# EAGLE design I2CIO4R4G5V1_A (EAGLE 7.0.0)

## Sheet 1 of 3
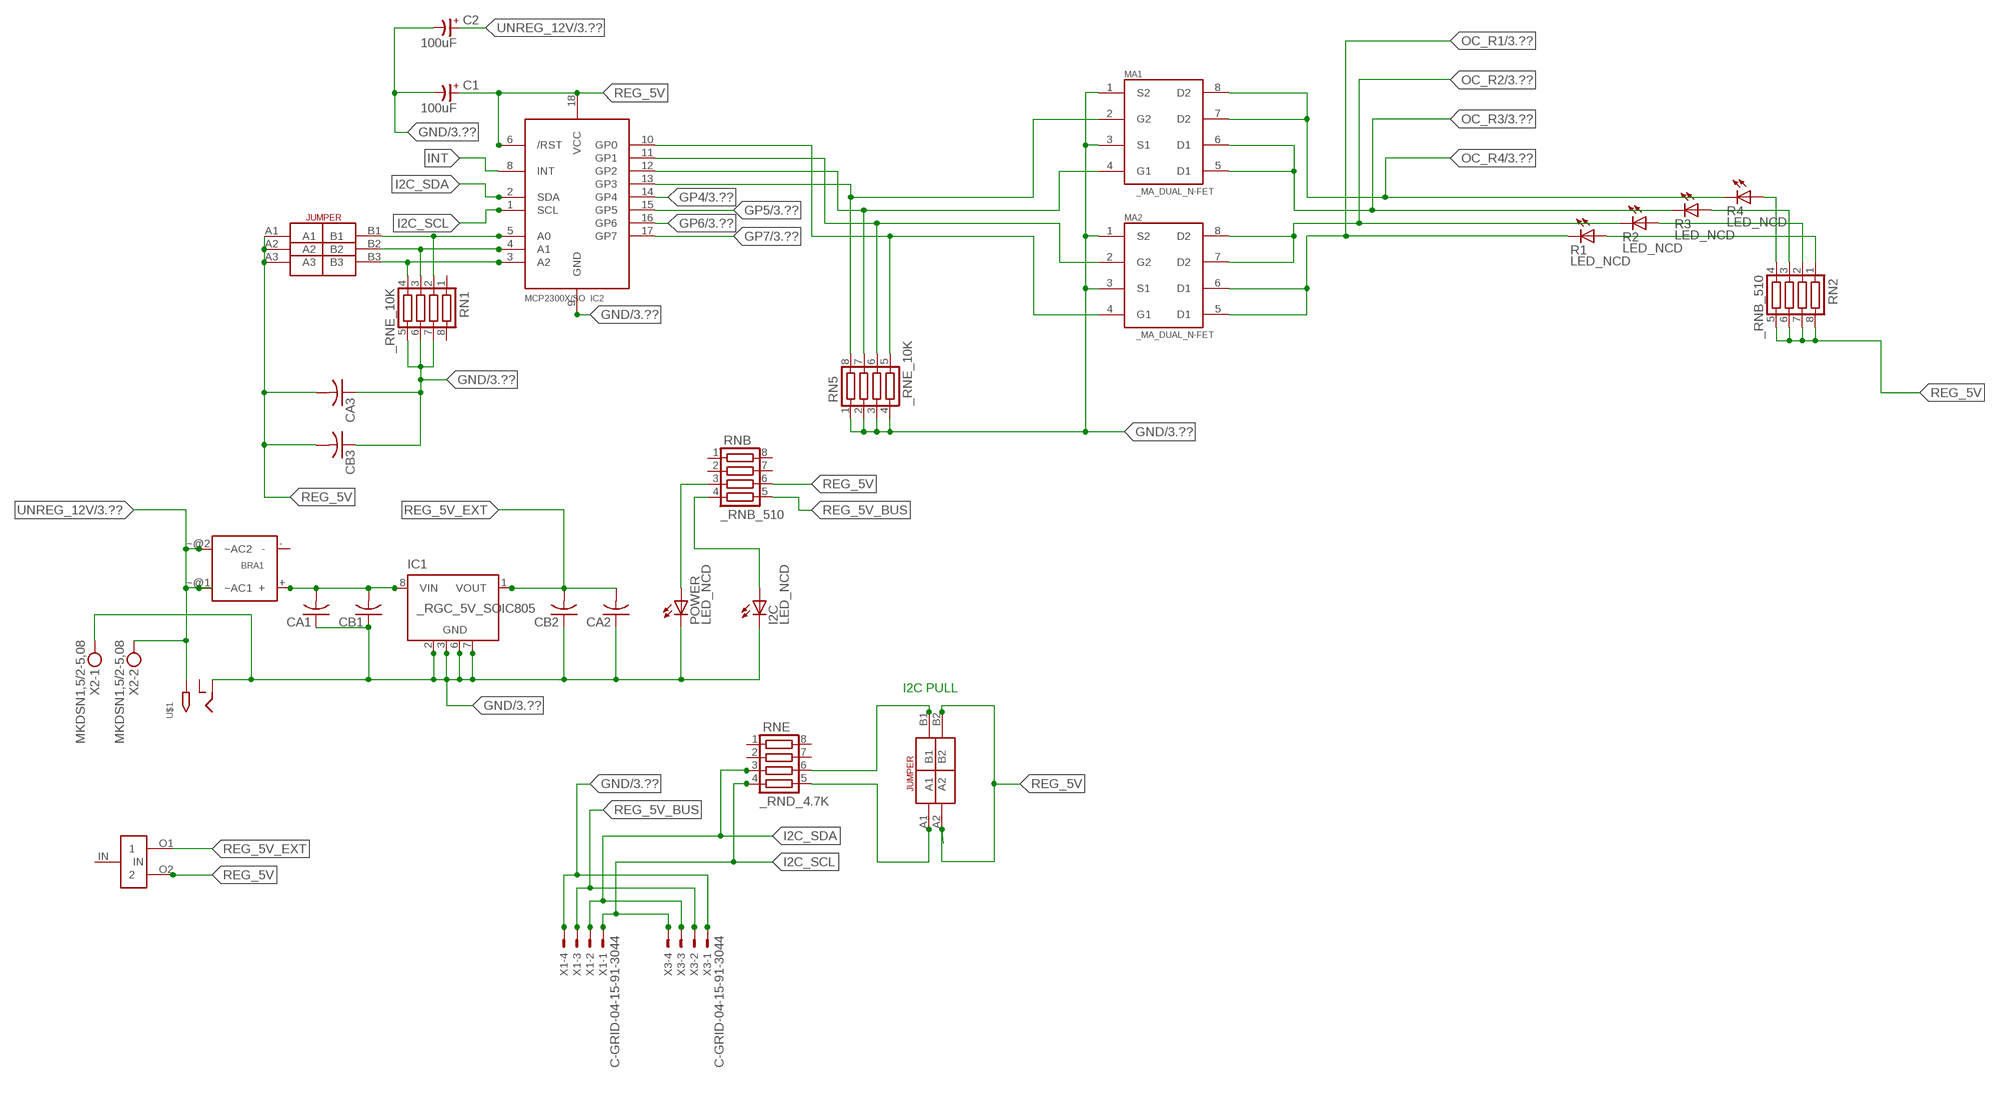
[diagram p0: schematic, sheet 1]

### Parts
BRA1  MB2S_  [MB2S]
C1  100uF  CP-E-025X060  [E-025X060]
C2  100uF  CP-E-025X060  [E-025X060]
CA1  CC1206KRX7R9BB104C1206K  [CC1206KRX7R9BB104]
CA2  CC1206KRX7R9BB104C1206K  [CC1206KRX7R9BB104]
CA3  CC1206KRX7R9BB104C1206K  [CC1206KRX7R9BB104]
CB1  TMK316F106ZL-TC1206K  [TMK316F106ZL-T]
CB2  TMK316F106ZL-TC1206K  [TMK316F106ZL-T]
CB3  TMK316F106ZL-TC1206K  [TMK316F106ZL-T]
I2C  LED_NCD  [CHIPLED_0603]
IC1  _RGC_5V_SOIC805  [_RGC_5V_SOIC8]
IC2  MCP2300X/SO  [SO18W]
MA1  _MA_DUAL_N-FET  [_MA_DUAL_N-FET]
MA2  _MA_DUAL_N-FET  [_MA_DUAL_N-FET]
POWER  LED_NCD  [CHIPLED_0603]
R1  LED_NCD  [CHIPLED_0603]
R2  LED_NCD  [CHIPLED_0603]
R3  LED_NCD  [CHIPLED_0603]
R4  LED_NCD  [CHIPLED_0603]
RN1  _RNE_10K  [RNE]
RN2  _RNB_510  [RNB]
RN5  _RNE_10K  [RNE]
RNB  _RNB_510  [RNB]
RNE  _RND_4.7K  [RND]
U$1  2.1MMJACK  [PJ-102A]
U$3  JUMPER_2X2  [JUMPER_2X2]
U$5  LINK_2  [LINK_2]
U$18  JUMPER_3X2  [JUMPER_3X2]
X1  C-GRID-04-15-91-3044  [15-91-04]
X2  MKDSN1,5/2-5,08  [MKDSN1,5/2-5,08]
X3  C-GRID-04-15-91-3044  [15-91-04]

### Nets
GND: C1.- C2.- CA1.1 CA2.1 CA3.1 CB1.1 CB2.1 CB3.1 I2C.C IC1.2(GND) IC1.3(GND) IC1.6(GND) IC1.7(GND) IC2.9(GND) MA1.1(S2) MA1.3(S1) MA2.1(S2) MA2.3(S1) POWER.C RN1.5 RN1.6 RN1.7 RN5.1 RN5.2 RN5.3 RN5.4 U$1.RING X1.4 X2.1 X3.1 ; also sheet 3
GP4: IC2.14(GP4) ; also sheet 3
GP5: IC2.15(GP5) ; also sheet 3
GP6: IC2.16(GP6) ; also sheet 3
GP7: IC2.17(GP7) ; also sheet 3
I2C_SCL: IC2.1(SCL) RNE.4 X1.1 X3.4
I2C_SDA: IC2.2(SDA) RNE.3 X1.2 X3.3
INT: IC2.8(INT)
N$1: BRA1.+ CA1.2 CB1.2 IC1.8(VIN)
N$2: POWER.A RNB.3
N$3: I2C.A RNB.4
N$4: RNE.5 U$3.A1
N$5: RNE.6 U$3.B1
N$6: IC2.5(A0) RN1.2 U$18.B1
N$7: IC2.4(A1) RN1.3 U$18.B2
N$8: IC2.3(A2) RN1.4 U$18.B3
N$20: IC2.13(GP3) MA1.2(G2) RN5.8
N$21: IC2.12(GP2) MA1.4(G1) RN5.7
N$22: IC2.11(GP1) MA2.2(G2) RN5.6
N$23: IC2.10(GP0) MA2.4(G1) RN5.5
N$29: R4.A RN2.4
N$30: R3.A RN2.3
N$31: R2.A RN2.2
N$32: R1.A RN2.1
OC_R1: MA2.5(D1) MA2.6(D1) R1.C ; also sheet 3
OC_R2: MA2.7(D2) MA2.8(D2) R2.C ; also sheet 3
OC_R3: MA1.5(D1) MA1.6(D1) R3.C ; also sheet 3
OC_R4: MA1.7(D2) MA1.8(D2) R4.C ; also sheet 3
REG_5V: C1.+ CA3.2 CB3.2 IC2.6(/RST) IC2.18(VCC) RN2.5 RN2.6 RN2.7 RN2.8 RNB.6 U$3.A2 U$3.B2 U$5.O2 U$18.A1 U$18.A2 U$18.A3
REG_5V_BUS: RNB.5 X1.3 X3.2
REG_5V_EXT: CA2.2 CB2.2 IC1.1(VOUT) U$5.O1
UNREG_12V: BRA1.~@1(~AC1) BRA1.~@2(~AC2) C2.+ U$1.TIP X2.2 ; also sheet 3
Unconnected: BRA1.- IC1.4(NC) IC1.5(NC) RN1.1 RN1.8 RNB.1 RNB.2 RNB.7 RNB.8 RNE.1 RNE.2 RNE.7 RNE.8 U$1.RING_SW U$5.IN

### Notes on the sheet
- I2C PULL

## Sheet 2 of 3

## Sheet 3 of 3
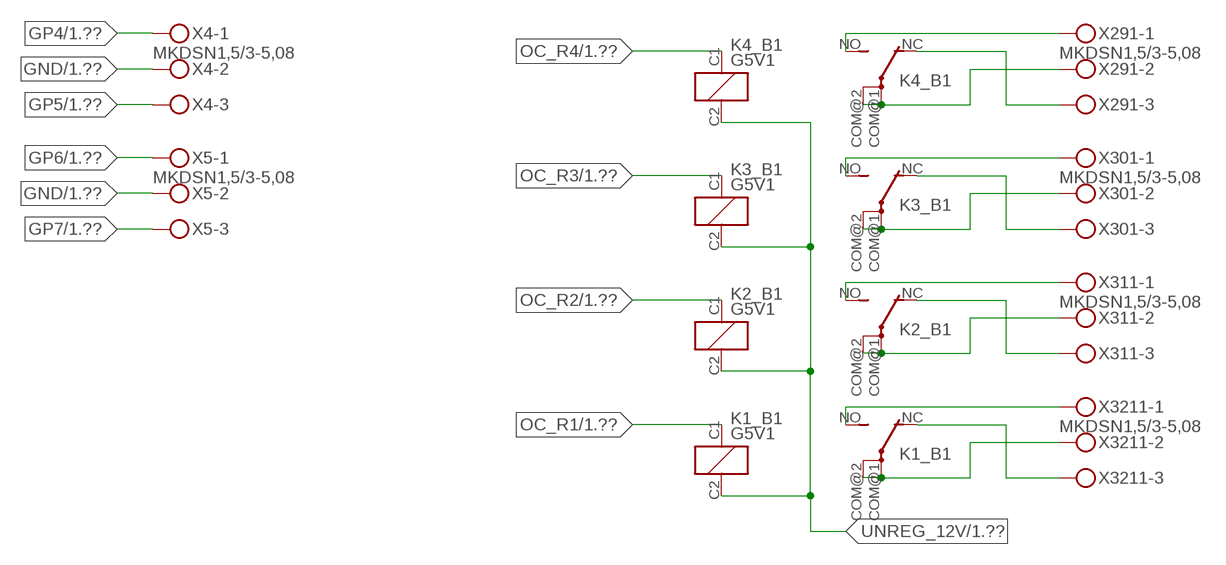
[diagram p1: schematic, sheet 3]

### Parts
K1_B1  G5V1  [G5V1]
K2_B1  G5V1  [G5V1]
K3_B1  G5V1  [G5V1]
K4_B1  G5V1  [G5V1]
X4  MKDSN1,5/3-5,08  [MKDSN1,5/3-5,08]
X5  MKDSN1,5/3-5,08  [MKDSN1,5/3-5,08]
X291  MKDSN1,5/3-5,08  [MKDSN1,5/3-5,08]
X301  MKDSN1,5/3-5,08  [MKDSN1,5/3-5,08]
X311  MKDSN1,5/3-5,08  [MKDSN1,5/3-5,08]
X3211  MKDSN1,5/3-5,08  [MKDSN1,5/3-5,08]

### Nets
GND: X4.2 X5.2 ; also sheet 1
GP4: X4.1 ; also sheet 1
GP5: X4.3 ; also sheet 1
GP6: X5.1 ; also sheet 1
GP7: X5.3 ; also sheet 1
N$215: K4_B1.NO(2:S) X291.1
N$216: K4_B1.NC(2:O) X291.3
N$217: K4_B1.COM@1(2:P) K4_B1.COM@2(2:P) X291.2
N$218: K3_B1.NO(2:S) X301.1
N$219: K3_B1.NC(2:O) X301.3
N$220: K3_B1.COM@1(2:P) K3_B1.COM@2(2:P) X301.2
N$221: K2_B1.NO(2:S) X311.1
N$222: K2_B1.NC(2:O) X311.3
N$223: K2_B1.COM@1(2:P) K2_B1.COM@2(2:P) X311.2
N$224: K1_B1.NO(2:S) X3211.1
N$225: K1_B1.NC(2:O) X3211.3
N$226: K1_B1.COM@1(2:P) K1_B1.COM@2(2:P) X3211.2
OC_R1: K1_B1.C1(1:C1) ; also sheet 1
OC_R2: K2_B1.C1(1:C1) ; also sheet 1
OC_R3: K3_B1.C1(1:C1) ; also sheet 1
OC_R4: K4_B1.C1(1:C1) ; also sheet 1
UNREG_12V: K1_B1.C2(1:C2) K2_B1.C2(1:C2) K3_B1.C2(1:C2) K4_B1.C2(1:C2) ; also sheet 1

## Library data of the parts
BRA1 = NCD_ULTIMATE_LIBRARY:MB2S: Bridge Rectifier BRA MB2S 200V 500ma Digikey MB2S-TPMSTR-ND/MB2S-TP
C1 C2 = NCD_ULTIMATE_LIBRARY:CP-: Capacitors All Kinds POLARIZED CAP
CA1-CA3 = NCD_ULTIMATE_LIBRARY:CC1206KRX7R9BB104: Capacitor CA .1uF 50V SMT C1206K CC1206KRX7R9BB104
CB1-CB3 = NCD_ULTIMATE_LIBRARY:TMK316F106ZL-T: Capacitor CB 10uF SMT 1206 TMK316F106ZL-T
I2C POWER = NCD_ULTIMATE_bhaskar:LED_NCD
IC1 = NCD_ULTIMATE_LIBRARY:_RGC_5V_SOIC8: Regulator Linear 5V Chip Positive VOLTAGE REGULATOR Digikey 497-7267-2-ND/L78L05CD13TR
IC2 = NCD_ULTIMATE_LIBRARY:MCP2300X: Semiconductor Port Expander I/O 8-Bit I2C MCP23008 Inexpensive i2c i/o expander - 8 general purpose i/o pins with optional pullups
K1_B1 K2_B1 K3_B1 K4_B1 = NCD_ULTIMATE_LIBRARY:G5V1: RELAY 1 x switch, 0.5 A/125 V AC, 1 A/24 V DC , Omron
MA1 MA2 = NCD_ULTIMATE_LIBRARY:_MA_DUAL_N-FET: FET Dual N-Channel 8-SOIC NMOSFET Digikey 785-1064-2-ND/AO4842
R1-R4 = NCD_ULTIMATE_LIBRARY:LED_NCD: LED Digikey 754-1132-2-ND/APT2012SRCPRV
RN1 RN5 = NCD_ULTIMATE_LIBRARY:_RNE_10K: Resistor Array RNE SMT 10K x 4 Single Resistor Source: http://www.ctscorp.com/components/Datasheets/CTSChipArrayDs.pdf Digikey 742C083103JPTR-ND/742C083103JP; OC_FARNELL: unknown; OC_NEWARK: unknown
RN2 RNB = NCD_ULTIMATE_LIBRARY:_RNB_510: Resistor Array RNB SMT 510 x 4 Single Resistor Source: http://www.ctscorp.com/components/Datasheets/CTSChipArrayDs.pdf Digikey 742C083511JPTR-ND/ 742C083511JP; OC_FARNELL: unknown; OC_NEWARK: unknown
RNE = NCD_ULTIMATE_LIBRARY:_RND_4.7K: Resistor Array RND SMT 4.7K x 4 Single Resistor Source: http://www.ctscorp.com/components/Datasheets/CTSChipArrayDs.pdf Digikey 742C083472JPTR-ND/742C083472JP; OC_FARNELL: unknown; OC_NEWARK: unknown
U$1 = NCD_ULTIMATE_CONNECTORS:2.1MMJACK: 2.1mm x 5.5mm DC jack with internal switch. Digikey part #PJ-102A, 4UCON part #05537 By microbuilder.eu
U$3 = NCD_ULTIMATE_CONNECTORS:JUMPER_2X2
U$5 = NCD_ULTIMATE_LIBRARY:LINK_2: PAD_top
U$18 = NCD_ULTIMATE_CONNECTORS:JUMPER_3X2
X1 X3 = NCD_ULTIMATE_CONNECTORS:C-GRID-04: CONNECTOR 4-Pos I2C wire to board 2.54 mm (0.100") pitch header Digikey WM1342-ND/0015912045; OC_FARNELL: unknown; OC_NEWARK: unknown
X2 = NCD_ULTIMATE_CONNECTORS:MKDSN1,5/2-5,08: MKDSN 1,5/ 2-5,08 Printklemme
X4 X5 X291 X301 X311 X3211 = NCD_ULTIMATE_CONNECTORS:MKDSN1,5/3-5,08: MKDSN 1,5/ 3-5,08 Printklemme Nennstrom: 13,5 A Nennspannung: 250 V Rastermaß: 5,08 mm Polzahl: 3 Anschlussart: Schraubanschluss Montage: Löten Anschlussrichtung Leiter/Platine: 0 ° Artikelnummer: 1729131 Source: http://eshop.phoenixcontact.com .. 1729131.pdf

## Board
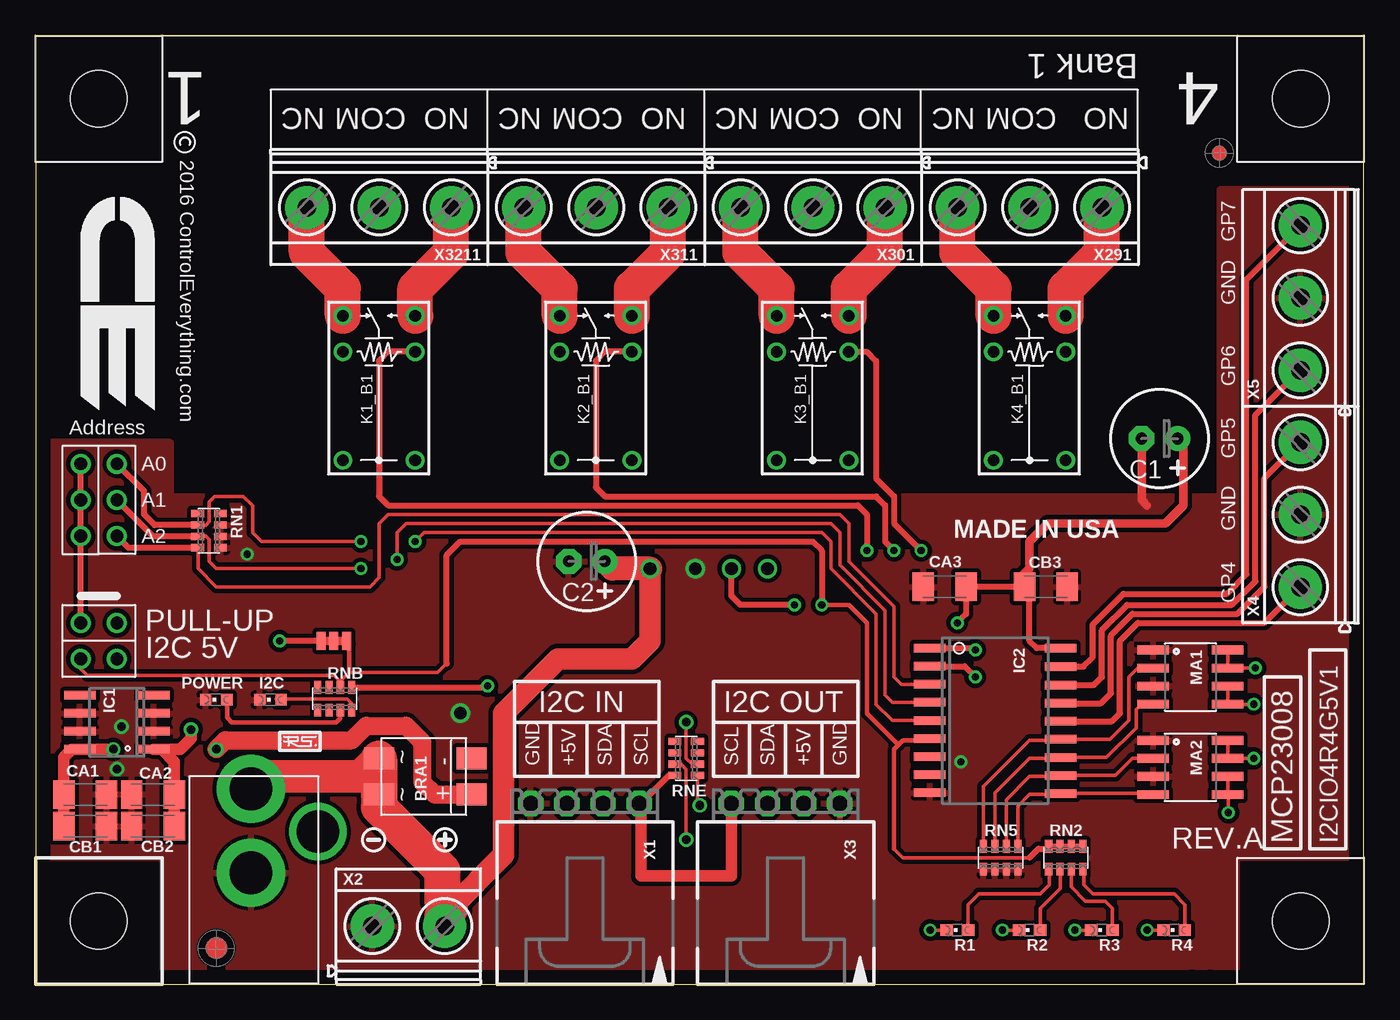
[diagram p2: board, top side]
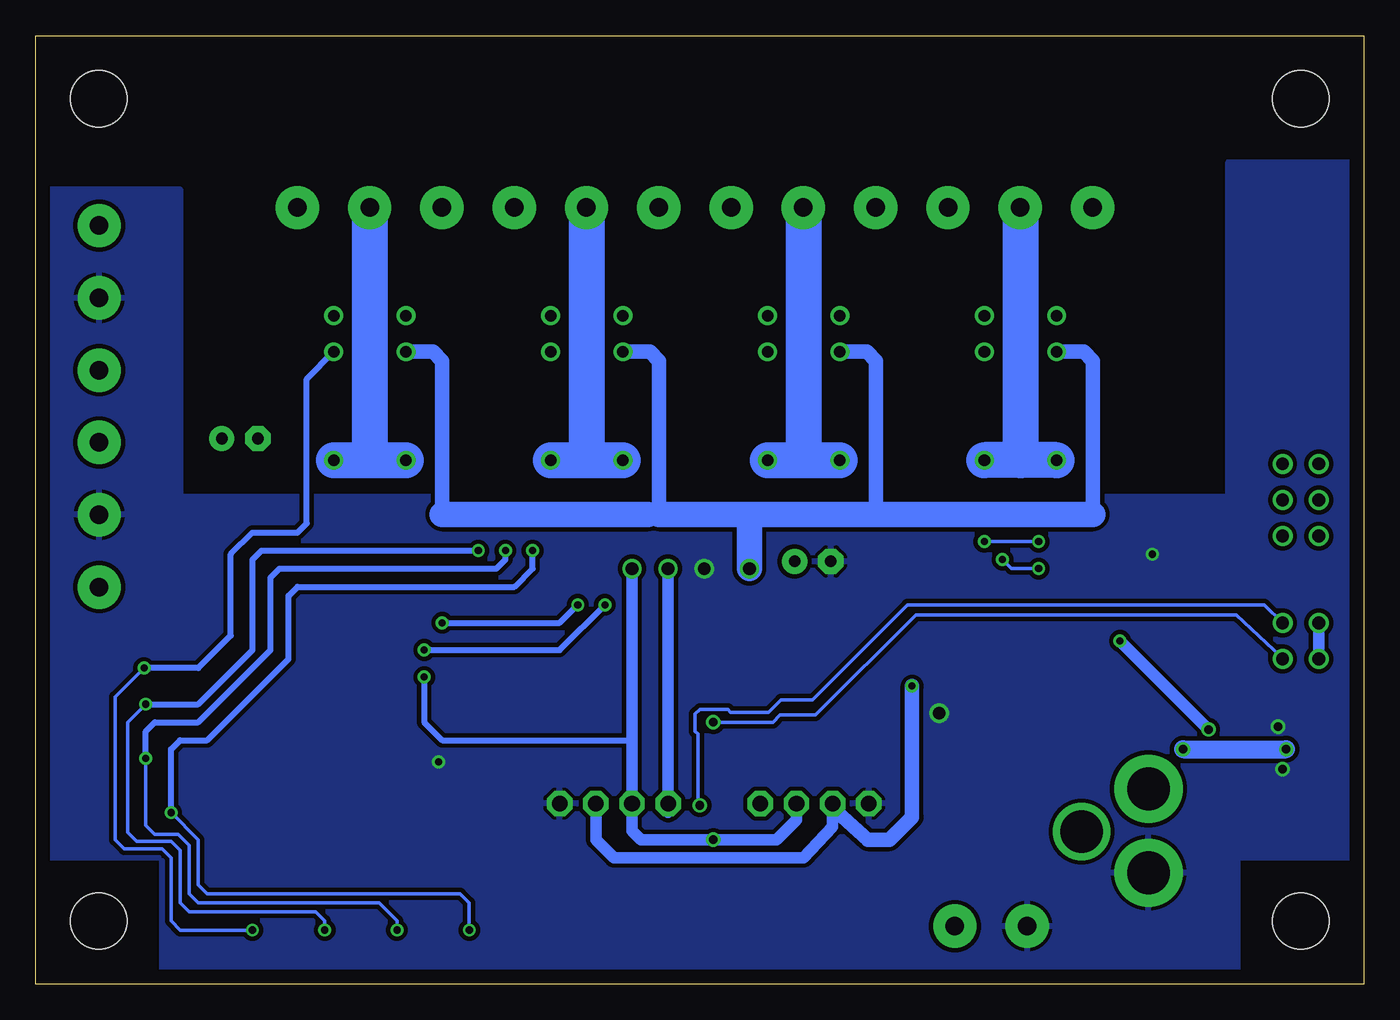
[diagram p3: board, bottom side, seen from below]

Size 93.34 x 66.67 mm. Coordinates in mm from the lower left corner, seen from the top.
Outline: 81.28,0 0,0 0,46.35
Outline: 81.28,0 82.53,0
Outline: 0,47.3 0,46.35
Outline: 81.28,0 93.34,0 93.34,66.67 0,66.67 0,46.35
Copper layers (1*16): Top 0.035mm / dielectric 1.5mm / Bottom 0.035mm
Design rules "default": minimum track width 10mil, minimum drill 24mil, track to track 8mil, track to pad 8mil, pad to pad 8mil, via to via 8mil, smd to smd 8mil, copper to edge 40mil, drill to drill 8mil, minimum pad ring 10mil, minimum via ring 8mil, stop-mask expansion 4mil, vias tented up to drill 0mil, thermal gap 10mil
Holes 3.96 mm at 4.45,4.45

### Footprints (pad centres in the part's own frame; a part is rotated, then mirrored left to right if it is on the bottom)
MB2S = smd 1.55 x 2.1: + 0,-6.5; - 2.54,-6.5; ~@1 0,0; ~@2 2.54,0
E-025X060 = drill 0.813 pad 1.778: + -1.27,0 | drill 0.813 pad 1.778 octagon: - 1.27,0
CC1206KRX7R9BB104 = smd 1.5 x 2: 1 -1.5,0; 2 1.5,0
TMK316F106ZL-T = smd 1.5 x 2: 1 -1.5,0; 2 1.5,0
CHIPLED_0603 = smd 0.8 x 0.8: A 0,-0.75; C 0,0.75
_RGC_5V_SOIC8 = smd 0.6 x 2.2: 1 -1.905,-2.6; 2 -0.635,-2.6; 3 0.635,-2.6; 4 1.905,-2.6; 5 1.905,2.6; 6 0.635,2.6; 7 -0.635,2.6; 8 -1.905,2.6
SO18W = smd 0.6 x 2.2: 1 -4.445,-4.6; 2 -3.175,-4.6; 3 -1.905,-4.6; 4 -0.635,-4.6; 5 0.635,-4.6; 6 1.905,-4.6; 7 3.175,-4.6; 8 4.445,-4.6; 9 5.715,-4.6; 10 5.775,4.6; 11 4.505,4.6; 12 3.235,4.6; 13 1.965,4.6; 14 0.695,4.6; 15 -0.575,4.6; 16 -1.845,4.6; 17 -3.145,4.6; 18 -4.445,4.6
G5V1 = drill 0.813: C1 -2.54,2.54; C2 -2.54,-2.54; COM@1 5.08,-2.54; COM@2 5.08,2.54; NC -5.08,-2.54; NO -5.08,2.54
_MA_DUAL_N-FET = smd 0.61 x 2.21: 1 -1.905,-2.616; 2 -0.635,-2.616; 3 0.635,-2.616; 4 1.905,-2.616; 5 1.905,2.616; 6 0.635,2.616; 7 -0.635,2.616; 8 -1.905,2.616
CHIPLED_0603' = smd 0.8 x 0.876: A 0,-0.75; C 0,0.75
RNE = smd 0.5 x 0.9: 1 -1.2,-0.8; 2 -0.4,-0.8; 3 0.4,-0.8; 4 1.2,-0.8; 5 1.2,0.8; 6 0.4,0.8; 7 -0.4,0.8; 8 -1.2,0.8
RNB = smd 0.5 x 0.9: 1 -1.2,-0.8; 2 -0.4,-0.8; 3 0.4,-0.8; 4 1.2,-0.8; 5 1.2,0.8; 6 0.4,0.8; 7 -0.4,0.8; 8 -1.2,0.8
RND = smd 0.5 x 0.9: 1 -1.2,-0.8; 2 -0.4,-0.8; 3 0.4,-0.8; 4 1.2,-0.8; 5 1.2,0.8; 6 0.4,0.8; 7 -0.4,0.8; 8 -1.2,0.8
PJ-102A = drill 3 pad 4.8: RING 0.1,-3.39; TIP 0.1,-9.29 | drill 3 pad 3.251: RING_SW -4.6,-6.29
JUMPER_2X2 = drill 0.9: A1 0,2.54; A2 0,0; B1 2.54,2.54; B2 2.54,0
PCB_MOUNTING_HOLE = hole 3.962: 4.445,4.445
LINK_2 = smd 1.27 x 0.635: IN 0,0; O1 0,0.889; O2 0,-0.889
JUMPER_3X2 = drill 0.9: A1 0,5.08; A2 0,2.54; A3 0,0; B1 2.54,5.08; B2 2.54,2.54; B3 2.54,0
15-91-04 = drill 1.1 pad 1.778 octagon: 1 -3.81,-7.62; 2 -1.27,-7.62; 3 1.27,-7.62; 4 3.81,-7.62
MKDSN1,5/2-5,08 = drill 1.3 pad 3.048: 1 -2.561,0.025; 2 2.519,0.025
MKDSN1,5/3-5,08 = drill 1.3 pad 3.048: 1 -7.641,0.025; 2 -2.561,0.025; 3 2.519,0.025

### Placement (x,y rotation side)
BRA1  24.13,13.34 90 top
C1  78.99,38.35 180 top
C2  38.73,29.72 180 top
CA1  3.49,13.34 180 top
CA2  8.26,13.34 0 top
CA3  63.88,27.94 0 top
CB1  3.49,11.11 180 top
CB2  8.26,11.11 0 top
CB3  70.99,27.94 180 top
I2C  16.51,20 90 top
IC1  5.71,18.41 90 top
IC2  67.44,19.18 270 top
K1_B1  24.13,41.91 270 top
K2_B1  39.37,41.91 270 top
K3_B1  54.61,41.91 270 top
K4_B1  69.85,41.91 270 top
MA1  81.15,21.59 270 top
MA2  81.15,15.24 270 top
POWER  12.7,20 90 top
R1  LED_NCD  [CHIPLED_0603']  64.77,3.81 90 top
R2  LED_NCD  [CHIPLED_0603']  69.85,3.81 90 top
R3  LED_NCD  [CHIPLED_0603']  74.93,3.81 90 top
R4  LED_NCD  [CHIPLED_0603']  80.01,3.81 90 top
RN1  12.19,31.88 270 top
RN2  72.39,8.89 0 top
RN5  67.82,8.89 0 top
RNB  21.02,20.07 0 top
RNE  45.72,15.88 270 top
U$1  15.24,4.45 180 top
U$3  3.17,25.4 270 top
U$4  PCB_MOUNTING_HOLE  [PCB_MOUNTING_HOLE]  93.34,57.78 90 top
U$5  20.95,24.13 90 top
U$6  PCB_MOUNTING_HOLE  [PCB_MOUNTING_HOLE]  93.34,0 90 top
U$10  [VISION_REF15]  12.7,2.54 0 top
U$11  PCB_MOUNTING_HOLE  [PCB_MOUNTING_HOLE]  8.89,57.78 90 top
U$18  3.17,31.5 0 top
U$19  [VISION_REF10]  83.19,58.42 0 top
U$21  [ICON_USA]  64.52,31.37 0 top
U$22  [ICON_MINUS]  23.75,10.16 180 top
U$24  [ICON_PLUS]  28.77,10.16 90 top
X1  38.61,5.08 180 top
X2  26.23,4.06 0 top
X3  52.7,5.08 180 top
X4  88.9,35.56 90 top
X5  88.9,50.8 90 top
X291  67.31,54.61 180 top
X301  52.07,54.61 180 top
X311  36.83,54.61 180 top
X3211  21.59,54.61 180 top

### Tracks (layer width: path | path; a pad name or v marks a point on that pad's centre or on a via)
GND  (via drill 0.5, 0.6, 0.9)
  Top 0.406: 34.8,12.38 X1.4
  Top 0.61: C1.- 77.72,34.04 78.11,33.66
  Top 0.813: X3.1 56.52,12.06
  other vias: 5.71,15.11 6.03,18.1 46.35,29.21 29.84,19.05 14.86,30.23 65.02,15.62
  pour Bottom (isolate 0.305): 0.64,8.89 8.89,8.89 8.89,0 84.45,0 84.45,8.89 92.71,8.89 92.71,55.88 83.19,55.88 83.19,34.29 9.53,34.29 9.53,57.78 0.64,57.78
  pour Top (isolate 0.305): -1.91,8.89 8.89,8.89 8.89,0 84.45,0 84.45,8.89 92.71,8.89 92.71,55.88 83.19,55.88 83.19,34.29 9.53,34.29 9.53,38.1 -1.91,38.1
GP4
  Top 0.406: IC2.14 75.63,18.48 76.2,19.05 76.2,24.13 77.47,25.4 86.36,25.4 X4.1
GP5
  Top 0.406: IC2.15 74.87,19.75 75.56,20.45 75.56,24.51 77.09,26.04 84.45,26.04 86.36,27.94 86.36,35.56 X4.3
GP6
  Top 0.406: IC2.16 74.36,21.02 74.93,21.59 74.93,24.89 76.71,26.67 84.07,26.67 85.72,28.32 85.72,40.01 X5.1
GP7
  Top 0.406: IC2.17 73.63,22.32 74.3,22.99 74.3,25.27 76.45,27.43 83.69,27.43 85.09,28.83 85.09,49.53 X5.3
I2C_SCL  (via drill 0.5, 0.9)
  Top 0.406: RNE.4 44.51,14.68 42.55,12.7 | IC2.1 65.91,23.62 v66.04,23.5 | v53.34,26.67 49.53,26.67 48.9,27.3 v48.9,29.21
  Top 0.813: X3.4 48.9,7.62 42.55,7.62 42.55,12.7 X1.1
  Bottom 0.406: v66.04,23.5 56.52,23.5 v53.34,26.67
  Bottom 0.813: v48.9,29.21 X3.4 48.9,12.06
I2C_SDA  (via drill 0.5, 0.6, 0.9)
  Top 0.254: RNE.3 45.36,15.47 45.72,15.11 v45.72,10.16
  Top 0.406: IC2.2 65.28,22.35 v66.04,21.59
  Top 0.61: X3.3 51.44,12.06 | X1.2 39.88,12.38
  Bottom 0.406: v66.04,21.59 66.04,18.41 64.77,17.14 51.44,17.14 | 39.88,12.38 X1.2
  Bottom 0.813: 39.88,12.38 39.88,11.56 41.27,10.16 v45.72,10.16 50.8,10.16 51.44,10.79 X3.3 51.44,17.14 v51.44,29.21
N$1  (via drill 0.6)
  Top 0.813: CB1.2 CA1.2 1.99,15.96 2.54,16.51 IC1.8 v5.46,16.51
  Top 1.27: v12.7,16.51 13.34,17.14 22.23,17.14 23.24,18.16 26.04,18.16 27.18,17.02 27.18,14.22 28.07,13.34 BRA1.+
  Bottom 1.27: v12.7,16.51 v5.46,16.51
N$2
  Top 0.305: RNB.3 21.4,18.95 21.4,18.7 21.12,18.41 13.78,18.41 13.45,18.74 POWER.A
N$3
  Top 0.254: 22.23,18.95 22.23,19.74 21.9,20.07 16.94,20.07
  Top 0.305: RNB.4 22.23,18.95 | 16.94,20.07 I2C.A
N$4  (via drill 0.6)
  Top 0.254: RNE.5 46.52,12.6 v46.67,12.57
  Bottom 0.254: U$3.A1 6.99,26.67 32.07,26.67 38.73,20 40.96,20 41.85,19.11 44.51,19.11 44.7,19.3 46.67,19.3 46.99,18.99 46.99,17.78 46.8,17.59 46.8,12.7 v46.67,12.57
N$5  (via drill 0.6)
  Top 0.254: RNE.6 46.12,15.47 45.72,15.88 v45.72,18.41
  Bottom 0.254: v45.72,18.41 41.53,18.41 41.02,18.92 38.54,18.92 31.5,25.97 8.95,25.97 6.35,23.5 U$3.B1
N$6  (via drill 0.5)
  Top 0.254: IC2.5 60.2,18.54 59.05,19.68 59.05,26.04 55.88,29.21 55.88,31.11 55.24,31.75 27.3,31.75 v26.67,31.11 | v22.86,31.11 15.88,31.11 15.24,31.75 15.24,33.66 14.61,34.29 12.57,34.29 12.19,33.91 12.19,32.51 11.94,32.26 11.41,32.26 RN1.2
  Top 0.406: RN1.2 8.36,32.28 7.62,33.02 7.62,34.67 U$18.B1
  Bottom 0.254: v26.67,31.11 v22.86,31.11
N$7  (via drill 0.5)
  Top 0.254: IC2.4 60.2,19.81 59.69,20.32 59.69,26.29 56.52,29.46 56.52,31.75 55.88,32.38 26.04,32.38 25.4,31.75 v25.4,29.84 | v22.86,29.21 12.7,29.21 12.19,29.72 12.19,31.24 11.94,31.5 11.41,31.5 RN1.3
  Top 0.406: RN1.3 8.27,31.48 U$18.B2
  Bottom 0.254: v25.4,29.84 24.77,29.21 v22.86,29.21
N$8
  Top 0.254: IC2.3 60.83,21.08 60.33,21.59 60.33,26.54 57.15,29.72 57.15,32.38 56.52,33.02 24.77,33.02 24.13,32.38 24.13,28.57 23.5,27.94 12.7,27.94 11.43,29.21 11.43,30.64 RN1.4
  Top 0.406: RN1.4 6.53,30.68 U$18.B3
N$20
  Top 0.254: MA1.2 77.47,22.23 76.83,21.59 76.83,18.54 75.5,17.21 IC2.13 71.97,17.14 69.85,17.14 66.62,13.91 RN5.8
N$21
  Top 0.254: MA1.4 77.72,19.68 77.34,19.3 77.34,18.03 75.25,15.94 IC2.12 71.97,15.88 69.85,15.88 67.42,13.44 RN5.7
N$22
  Top 0.254: MA2.2 77.09,15.88 75.89,14.67 IC2.11 71.97,14.61 69.85,14.61 68.22,12.97 RN5.6
N$23
  Top 0.254: MA2.4 78.6,13.4 IC2.10 71.97,13.34 69.85,13.34 69.02,12.5 RN5.5
N$29
  Top 0.254: R4.A 80.76,5.6 80.01,6.35 74.3,6.35 73.66,6.99 73.66,8.02 RN2.4
N$30
  Top 0.254: R3.A 75.68,5.35 75.18,5.84 73.79,5.84 72.77,6.86 72.77,8.07 RN2.3
N$31
  Top 0.254: R2.A 70.6,5.32 72.01,6.73 72.01,8.07 RN2.2
N$32
  Top 0.254: R1.A 65.52,5.58 66.29,6.35 70.61,6.35 71.25,6.99 71.25,8.03 RN2.1
N$215
  Top 2.54: K4_B1.NO 72.39,48.9 74.93,51.44 74.93,54.56 X291.1
N$216
  Top 2.54: K4_B1.NC 67.31,48.9 64.77,51.44 64.77,54.56 X291.3
N$217
  Bottom 2.54: X291.2 69.87,36.85 | 69.87,36.85 69.85,36.83 K4_B1.COM@1 | K4_B1.COM@2 69.89,36.83 69.87,36.85
N$218
  Top 2.54: K3_B1.NO 57.15,48.9 59.69,51.44 59.69,54.56 X301.1
N$219
  Top 2.54: K3_B1.NC 52.07,48.9 49.53,51.44 49.53,54.56 X301.3
N$220
  Bottom 2.54: K3_B1.COM@2 54.61,36.83 | 54.61,36.83 K3_B1.COM@1 | X301.2 54.63,36.85 54.61,36.83
N$221
  Top 2.54: K2_B1.NO 41.91,48.9 44.45,51.44 44.45,54.56 X311.1
N$222
  Top 2.54: K2_B1.NC 36.83,48.9 34.29,51.44 34.29,54.56 X311.3
N$223
  Bottom 2.54: K2_B1.COM@2 39.37,36.83 | 39.37,36.83 K2_B1.COM@1 | X311.2 39.39,36.85 39.37,36.83
N$224
  Top 2.54: K1_B1.NO 26.67,48.9 29.21,51.44 29.21,54.56 X3211.1
N$225
  Top 2.54: K1_B1.NC 21.59,48.9 19.05,51.44 19.05,54.56 X3211.3
N$226
  Bottom 2.54: K1_B1.COM@1 24.13,36.83 | 24.13,36.83 K1_B1.COM@2 | X3211.2 24.15,36.85 24.13,36.83
OC_R1  (via drill 0.5)
  Top 0.254: R1.C v62.87,3.81 | v83.82,12.06 83.82,13.26 MA2.5 MA2.6
  Top 0.406: v58.42,30.48 58.42,33.02 57.78,33.66 24.77,33.66 24.13,34.29 24.13,43.81 24.77,44.45 K1_B1.C1
  Bottom 0.254: v62.87,3.81 62.87,5.71 63.5,6.35 81.28,6.35 81.92,6.99 81.92,10.16 v83.82,12.06
  Bottom 0.406: v83.82,12.06 83.82,16.51 83.19,17.14 81.28,17.14 75.56,22.86 75.56,27.3 74.93,27.94 59.69,27.94 58.42,29.21 v58.42,30.48
OC_R2  (via drill 0.5)
  Top 0.254: R2.C v67.94,3.81 | v85.6,15.88 MA2.7 MA2.8
  Top 0.406: v60.33,30.48 59.69,31.11 59.69,33.66 59.05,34.29 40.01,34.29 39.37,34.92 39.37,43.81 40.01,44.45 K2_B1.C1
  Bottom 0.254: v67.94,3.81 67.94,4.45 69.22,5.71 81.92,5.71 82.55,6.35 82.55,9.78 83.31,10.54 84.96,10.54 85.6,11.18 v85.6,15.88
  Bottom 0.406: v85.6,15.88 85.6,17.78 84.96,18.41 81.92,18.41 76.83,23.5 76.83,28.57 76.2,29.21 60.96,29.21 60.33,29.84 v60.33,30.48
OC_R3  (via drill 0.5)
  Top 0.254: R3.C v73.03,3.81 | v85.6,19.68 MA1.5 MA1.6
  Top 0.406: 61.85,30.86 v62.23,30.48 60.33,32.38 60.33,34.29 59.05,35.56 59.05,43.81 58.42,44.45 K3_B1.C1
  Bottom 0.254: v73.03,3.81 73.03,4.45 73.66,5.08 82.55,5.08 83.19,5.71 83.19,9.4 83.82,10.03 86.23,10.03 86.87,10.67 86.87,18.41 v85.6,19.68
  Bottom 0.406: v85.6,19.68 81.92,19.68 78.11,23.5 78.11,29.84 77.47,30.48 v62.23,30.48
OC_R4  (via drill 0.5)
  Top 0.254: R4.C v78.11,3.81 | v85.72,22.23 MA1.7 MA1.8
  Bottom 0.254: v78.11,3.81 83.19,3.81 83.82,4.45 83.82,8.89 84.45,9.53 87.12,9.53 87.76,10.16 87.76,20.19 v85.72,22.23
  Bottom 0.406: v85.72,22.23 81.92,22.23 79.63,24.51 79.63,30.23 78.11,31.75 74.93,31.75 74.3,32.38 74.3,42.55 K4_B1.C1
REG_5V  (via drill 0.5)
  Top 0.229: 60.33,9.53 60.96,8.89 69.85,8.89
  Top 0.254: RNB.6 21.42,21.29 | 21.42,21.29 22.04,21.91 28.26,21.91 28.89,22.54 | 21.42,21.29 20.99,21.72 3.62,21.72 3.17,22.16 U$3.B2
  Top 0.305: 62.71,17.14 60.96,17.14 60.64,16.83 | 60.64,16.83 60.33,16.51 60.33,9.53 | 60.64,16.83 58.42,19.05 58.42,25.4 57.15,26.67 v55.24,26.67 | 22.04,21.91 22.04,23.94 U$5.O2
  Top 0.406: U$18.A1 U$18.A2 U$18.A3 U$3.A2 | IC2.18 70.36,23.62 69.85,24.13 69.85,27.58 CB3.2 CA3.2 65.38,26.01 v64.77,25.4 | 62.71,17.14 IC2.6 | 69.85,8.89 70.48,9.53 71.03,9.53 RN2.8 RN2.7 RN2.6 RN2.5 | 28.89,22.54 28.89,30.16 29.84,31.11 54.61,31.11 55.24,30.48 v55.24,26.67
  Top 0.61: CB3.2 69.22,28.22 69.22,28.57 69.85,29.21 69.85,31.11 71.12,32.38 79.38,32.38 80.64,33.66 80.64,37.97 C1.+
  Bottom 0.406: v64.77,25.4 56.52,25.4 v55.24,26.67
  Bottom 0.813: U$3.B2 U$3.A2
REG_5V_BUS  (via drill 0.5)
  Top 0.406: RNB.5 31.66,20.87 v31.75,20.95
  Top 0.61: X1.3 37.34,12.38 | X3.2 53.98,12.06
  Bottom 0.406: 37.34,12.38 X1.3 | 53.98,12.06 X3.2
  Bottom 0.813: 37.34,12.38 37.34,11.05 39.37,8.89 52.7,8.89 53.98,10.16 53.98,12.06
  Bottom 1.016: 37.34,12.38 34.86,10.16 33.34,10.16 31.75,11.75 v31.75,20.95
REG_5V_EXT  (via drill 0.5, 0.6)
  Top 0.406: U$5.O1 v17.14,24.13
  Top 0.813: CB2.2 CA2.2 9.76,15.64 8.89,16.51 | 8.89,16.51 IC1.1 | v10.92,17.91 10.92,17.27 10.16,16.51 8.89,16.51
  Bottom 0.813: v17.14,24.13 v10.92,17.91
UNREG_12V  (via drill 0.9)
  Top 1.524: v43.18,29.21 43.18,24.13 41.91,22.86 36.7,22.86 32.89,19.05 32.89,9.08 29.11,5.3 28.57,4.76
  Top 1.676: v43.18,29.21 40.51,29.21 C2.+
  Top 2.286: BRA1.~@2 22.86,14.61 16.01,14.61
  Top 2.54: 16.01,14.61 U$1.TIP | X2.2 28.55,4.45 28.57,4.76 | BRA1.~@2 BRA1.~@1 24.13,12.45 28.57,8 28.57,5.84 29.11,5.3
  Bottom 1.016: K4_B1.C2 65.41,44.45 64.77,43.81 64.77,33.02 | K3_B1.C2 50.16,44.45 49.53,43.81 49.53,33.15 | 49.53,33.15 50.29,33.02 | 49.53,33.15 49.66,33.15 49.53,33.02 | K2_B1.C2 34.92,44.45 34.29,43.81 34.29,33.02 | K1_B1.C2 19.68,44.45 19.05,43.81 19.05,33.02
  Bottom 1.778: v43.18,29.21 43.18,33.02 | 43.18,33.02 34.29,33.02 19.05,33.02 | 49.53,33.02 43.18,33.02 | 64.77,33.02 50.29,33.02

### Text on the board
tNames: Bank 1 | 1 | 4 | NC | COM | NO | NC | COM | NO | NC | COM | NO | NC | COM | NO | 2016 ControlEverything.com | GP7 | GND | GP6 | Address | GP5 | A0 | A1 | GND | A2 | GP4 | PULL-UP | I2C 5V | I2C IN | I2C OUT | GND | +5V | SDA | SCL | SCL | SDA | +5V | +5V | GND | REV.A | MCP23008 | I2CIO4R4G5V1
